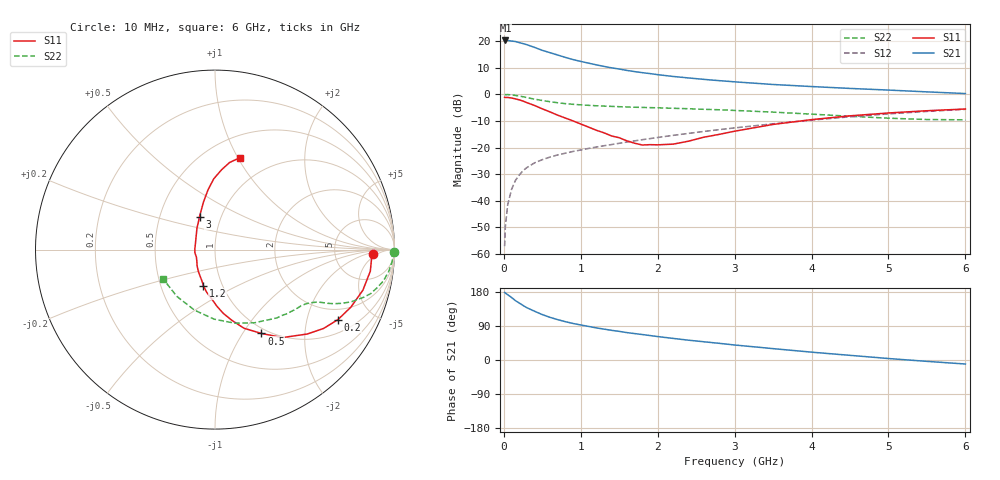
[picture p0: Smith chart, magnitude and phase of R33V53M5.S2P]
! SIEMENS Small Signal Semiconductors
! BFR181
! Si NPN RF Bipolar Junction Transistor in SOT23
! VCE = 3.5 V  IC = 3.5 mA
! Common Emitter S-Parameters:  May  1996
# GHz  S  MA  R  50
!  f  S11  S21  S12  S22
! GHz  MAG  ANG  MAG  ANG  MAG  ANG  MAG  ANG
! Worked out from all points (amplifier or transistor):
!   36 points, 10 MHz to 6 GHz, reference 50 ohm
!   highest |S21| = 20.3 dB at 20 MHz (marker M1)
!   |S21| within 3 dB of that: start of sweep to 434.6 MHz
!   unconditionally stable (mu >= 1): 1.292 GHz to 3.128 GHz
!   at 250 MHz: K = 0.33, MSG = 23.9 dB, |S12| = -28.7 dB
!   at 1.4 GHz: K = 1.02, MAG = 13.5 dB, |S12| = -18.9 dB
!   at 6 GHz: K = 0.86, MSG = 3.0 dB, |S12| = -5.6 dB
!   S11 on the Smith chart (normalised r, x): 10 MHz: 15, -3; 200 MHz: 1.50, -3.10; 500 MHz: 0.93, -1.22; 1.2 GHz: 0.81, -0.34; 3 GHz: 0.79, +0.30; 6 GHz: 0.72, +1.02
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0.01  0.8795 -1.7  10.26 178.4  0.0014 95.0  0.9946 -0.7
0.02  0.8737 -3.3  10.3 176.6  0.0033 85.5  0.9866 -1.5
0.05  0.8737 -7.9  10.29 172.2  0.0084 85.6  0.9898 -3.7
0.15  0.8224 -22.9  9.859 156.7  0.024 77.6  0.954 -10.6
0.2  0.788 -29.7  9.392 150.4  0.0304 73.6  0.9272 -13.3
0.25  0.7475 -36.0  8.989 143.9  0.0368 70.8  0.9013 -15.8
0.3  0.6973 -42.4  8.57 137.9  0.0421 69.0  0.8692 -17.8
0.4  0.6171 -52.6  7.623 128.6  0.0516 64.7  0.8127 -21.0
0.5  0.5342 -61.0  6.713 119.8  0.0592 62.2  0.766 -23.0
0.6  0.4675 -69.7  6.069 112.6  0.0662 60.8  0.7272 -24.5
0.7  0.4059 -76.5  5.487 106.5  0.0727 60.3  0.6949 -25.5
0.8  0.3582 -82.6  4.947 101.1  0.0783 59.5  0.6692 -26.2
0.9  0.3163 -88.0  4.503 96.4  0.0845 59.7  0.6495 -26.8
1.1  0.2428 -100.9  3.863 88.7  0.0962 59.9  0.6219 -28.3
1.2  0.2119 -107.7  3.593 84.8  0.1021 60.4  0.6108 -29.0
1.6  0.1336 -138.4  2.815 72.3  0.127 60.9  0.5796 -32.2
2.2  0.1158 159.4  2.169 57.0  0.1695 60.8  0.547 -39.0
3  0.2028 115.2  1.719 39.6  0.2341 57.2  0.4983 -51.1
3.5  0.272 103.7  1.532 30.0  0.2794 53.8  0.4634 -61.6
4.5  0.3945 91.0  1.292 12.3  0.3786 44.2  0.3874 -90.8
5.5  0.4919 80.5  1.113 -3.6  0.4779 31.7  0.3364 -129.0
6  0.5304 74.9  1.035 -10.6  0.5229 24.6  0.3318 -150.2
